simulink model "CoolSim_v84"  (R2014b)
settings: Solver=ode1  StartTime=0.0  StopTime=trun  FixedStep=dtmax  MaxStep=dtmax  MinStep=1e-6  RelTol=1e-4
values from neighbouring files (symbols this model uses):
  aperp_cond = l_cond*gappl_cond - l_cond*densfin_cond*thfin_cond*lfin_cond    (= 0.00397716486616)    [CoolSim_v84_ec_init.m]    (also in CoolSim_v84_mc_init.m)
  apin_txv = 1e-3^2/4*pi    (= 7.85398163397e-07)    [CoolSim_v84_ec_init.m]    (also in CoolSim_v84_mc_init.m)
  area_cabinint = 8.0    (= 8)    [CoolSim_v84_ec_init.m]    (also in CoolSim_v84_mc_init.m)
  area_cabinshell = 4.0    (= 4)    [CoolSim_v84_ec_init.m]    (also in CoolSim_v84_mc_init.m)
  aseat_txv = dball_txv^2/4*pi    (= 7.06858347058e-06)    [CoolSim_v84_ec_init.m]    (also in CoolSim_v84_mc_init.m)
  atop_txv = 400e-6    (= 0.0004)    [CoolSim_v84_ec_init.m]    (also in CoolSim_v84_mc_init.m)
  c08 = -5.8002206e+003    (= -5800.2206)    [CoolSim_v84_ec_init.m]    (also in CoolSim_v84_mc_init.m)
  c09 = 1.3914993    [CoolSim_v84_ec_init.m]    (also in CoolSim_v84_mc_init.m)
  c10 = -4.8640239E-02    (= -0.048640239)    [CoolSim_v84_ec_init.m]    (also in CoolSim_v84_mc_init.m)
  c11 = 4.1764768E-05    (= 4.1764768e-05)    [CoolSim_v84_ec_init.m]    (also in CoolSim_v84_mc_init.m)
  c12 = -1.4452093E-08    (= -1.4452093e-08)    [CoolSim_v84_ec_init.m]    (also in CoolSim_v84_mc_init.m)
  c13 = 6.5459673    [CoolSim_v84_ec_init.m]    (also in CoolSim_v84_mc_init.m)
  c1_comprmech = 0.8728    [CoolSim_v84_ec_init.m]    (also in CoolSim_v84_mc_init.m = 0.9)
  c2_comprmech = 0.1777    [CoolSim_v84_ec_init.m]    (also in CoolSim_v84_mc_init.m = 0)
  cv_air = 719.    (= 719)    [CoolSim_v84_ec_init.m]    (also in CoolSim_v84_mc_init.m)
  deltat = 2e-4    (= 0.0002)    [CoolSim_v84_ec_init.m]    (also in CoolSim_v84_mc_init.m)
  dh_evaptocomp = 0.0    (= 0)    [CoolSim_v84_ec_init.m]    (also in CoolSim_v84_mc_init.m)
  displ_compr = 33e-6    (= 3.3e-05)    [CoolSim_v84_ec_init.m]    (also in CoolSim_v84_mc_init.m = 0.0002)
  dp_blower = [0,  40., 160., 360.]    [CoolSim_v84_ec_init.m]    (also in CoolSim_v84_mc_init.m)
  dp_evaptocomp = 0.0    (= 0)    [CoolSim_v84_ec_init.m]    (also in CoolSim_v84_mc_init.m)
  dpair_cond = 2300.    (= 2300)    [CoolSim_v84_ec_init.m]    (also in CoolSim_v84_mc_init.m)
  dt_evapout = 0.5    [CoolSim_v84_ec_init.m]    (also in CoolSim_v84_mc_init.m)
  dt_thermostat = 0.2    [CoolSim_v84_ec_init.m]    (also in CoolSim_v84_mc_init.m)
  eff_blower = 0.12    [CoolSim_v84_ec_init.m]    (also in CoolSim_v84_mc_init.m)
  eff_fan = 0.15    [CoolSim_v84_ec_init.m]    (also in CoolSim_v84_mc_init.m)
  einitvec_cond1 = 10.*ones(1,nseg_cond1)    [CoolSim_v84_ec_init.m]    (also in CoolSim_v84_mc_init.m)
  einitvec_cond2 = 10.*ones(1,nseg_cond2)    [CoolSim_v84_ec_init.m]    (also in CoolSim_v84_mc_init.m)
  einitvec_evap1 = 10.*ones(1,nseg_evap1)    [CoolSim_v84_ec_init.m]    (also in CoolSim_v84_mc_init.m)
  einitvec_evap2a = 10.*ones(1,nseg_evap2)    [CoolSim_v84_ec_init.m]    (also in CoolSim_v84_mc_init.m)
  einitvec_evap2b = 10.*ones(1,nseg_evap2)    [CoolSim_v84_ec_init.m]    (also in CoolSim_v84_mc_init.m)
  einitvec_evap3 = 10.*ones(1,nseg_evap3)    [CoolSim_v84_ec_init.m]    (also in CoolSim_v84_mc_init.m)
  einitvec_evap4 = 10.*ones(1,nseg_evap4)    [CoolSim_v84_ec_init.m]    (also in CoolSim_v84_mc_init.m)
  f1_blowcontr = -0.7    [CoolSim_v84_ec_init.m]    (also in CoolSim_v84_mc_init.m)
  f1_comprcontr = -0.02    [CoolSim_v84_ec_init.m]    (also in CoolSim_v84_mc_init.m)
  f2_blowcontr = 0.005    [CoolSim_v84_ec_init.m]    (also in CoolSim_v84_mc_init.m)
  f2_comprcontr = 1./6.    (= 0.166666666667)    [CoolSim_v84_ec_init.m]    (also in CoolSim_v84_mc_init.m)
  fp_txv = (psetbulb_txv - pset_txv)*atop_txv - 15e5*aseat_txv    [CoolSim_v84_ec_init.m]    (also in CoolSim_v84_mc_init.m)
  h_lookuphvsps = h1    [CoolSim_v84_ec_init.m]    (also in CoolSim_v84_mc_init.m)
  hmax_heater = 8000.    (= 8000)    [CoolSim_v84_ec_init.m]    (also in CoolSim_v84_mc_init.m)
  htin_enginecomp = 0.0    (= 0)    [CoolSim_v84_ec_init.m]    (also in CoolSim_v84_mc_init.m; point_ec01.m; point_mc01.m)
  htin_solarintvstime = [htin_solarint htin_solarint]    [CoolSim_v84_ec_init.m]    (also in CoolSim_v84_mc_init.m; point_ec01.m = [300. 300.]; point_mc01.m = [300. 300.])
  htin_solarshellvstime = [htin_solarshell htin_solarshell]    [CoolSim_v84_ec_init.m]    (also in CoolSim_v84_mc_init.m; point_ec01.m = [1000. 1000.]; point_mc01.m = [1000. 1000.])
  htrans_cabinint = 25.    (= 25)    [CoolSim_v84_ec_init.m]    (also in CoolSim_v84_mc_init.m)
  htrans_cabinshell = 15.    (= 15)    [CoolSim_v84_ec_init.m]    (also in CoolSim_v84_mc_init.m)
  ifmech = 0.0    (= 0)    [CoolSim_v84_ec_init.m]    (also in CoolSim_v84_mc_init.m = 1)
  iinitvec_cond1 = 0.0*ones(1,nseg_cond1+1)    [CoolSim_v84_ec_init.m]    (also in CoolSim_v84_mc_init.m)
  iinitvec_cond2 = 0.0*ones(1,nseg_cond2+1)    [CoolSim_v84_ec_init.m]    (also in CoolSim_v84_mc_init.m)
  iinitvec_evap1 = 0.0*ones(1,nseg_evap1+1)    [CoolSim_v84_ec_init.m]    (also in CoolSim_v84_mc_init.m)
  iinitvec_evap2a = 0.0*ones(1,nseg_evap2+1)    [CoolSim_v84_ec_init.m]    (also in CoolSim_v84_mc_init.m)
  iinitvec_evap2b = 0.0*ones(1,nseg_evap2+1)    [CoolSim_v84_ec_init.m]    (also in CoolSim_v84_mc_init.m)
  iinitvec_evap3 = 0.0*ones(1,nseg_evap3+1)    [CoolSim_v84_ec_init.m]    (also in CoolSim_v84_mc_init.m)
  iinitvec_evap4 = 0.0*ones(1,nseg_evap4+1)    [CoolSim_v84_ec_init.m]    (also in CoolSim_v84_mc_init.m)
  init_memrestart = 2250.    (= 2250)    [CoolSim_v84_ec_init.m]    (also in CoolSim_v84_mc_init.m; reinit.m = memrestart(n,2))
  init_picontr1 = 0.23    [CoolSim_v84_ec_init.m]    (also in CoolSim_v84_mc_init.m; reinit.m = picontr1(n,2))
  init_picontr2 = 0.32    [CoolSim_v84_ec_init.m]    (also in CoolSim_v84_mc_init.m; reinit.m = picontr2(n,2))
  iseff_rpm_pr = [0.650   0.728   0.717   0.655   0.569;     0.570   0.682   0.700   0.637   0.536;     0.460   0.590   0.650   0.600   0.493;     0.290   0.496   0.618   0.575   0.450]    [CoolSim_v84_ec_init.m]    (also in CoolSim_v84_mc_init.m = [0.8490    0.8490    0.7829    0.7409    0.7065    0.6802   )
  k_cabinleakin = 1e-4    (= 0.0001)    [CoolSim_v84_ec_init.m]    (also in CoolSim_v84_mc_init.m)
  k_cabinleakout = 4e-4    (= 0.0004)    [CoolSim_v84_ec_init.m]    (also in CoolSim_v84_mc_init.m)
  k_ram = 0.1    [CoolSim_v84_ec_init.m]    (also in CoolSim_v84_mc_init.m)
  l_cabinsurf = 2.0    (= 2)    [CoolSim_v84_ec_init.m]    (also in CoolSim_v84_mc_init.m)
  md_comprmax = rpm_max/60.*displ_compr*0.975*27.8    (= 0.10435425)    [CoolSim_v84_ec_init.m]    (also in CoolSim_v84_mc_init.m = 0.63245)
  minitvec_cond1 = 1e-4*ones(1,nseg_cond1)    [CoolSim_v84_ec_init.m]    (also in CoolSim_v84_mc_init.m)
  minitvec_cond2 = 1e-4*ones(1,nseg_cond2)    [CoolSim_v84_ec_init.m]    (also in CoolSim_v84_mc_init.m)
  minitvec_evap1 = 1e-4*ones(1,nseg_evap1)    [CoolSim_v84_ec_init.m]    (also in CoolSim_v84_mc_init.m)
  minitvec_evap2a = 1e-4*ones(1,nseg_evap2)    [CoolSim_v84_ec_init.m]    (also in CoolSim_v84_mc_init.m)
  minitvec_evap2b = 1e-4*ones(1,nseg_evap2)    [CoolSim_v84_ec_init.m]    (also in CoolSim_v84_mc_init.m)
  minitvec_evap3 = 1e-4*ones(1,nseg_evap3)    [CoolSim_v84_ec_init.m]    (also in CoolSim_v84_mc_init.m)
  minitvec_evap4 = 1e-4*ones(1,nseg_evap4)    [CoolSim_v84_ec_init.m]    (also in CoolSim_v84_mc_init.m)
  mrefr_outrate = 0.2    [CoolSim_v84_ec_init.m]    (also in CoolSim_v84_mc_init.m)
  mrefr_targ = 0.48    [CoolSim_v84_ec_init.m]    (also in CoolSim_v84_mc_init.m)
  nc1 = 35.    (= 35)    [CoolSim_v84_ec_init.m]    (also in CoolSim_v84_mc_init.m)
  nc2 = 9.0    (= 9)    [CoolSim_v84_ec_init.m]    (also in CoolSim_v84_mc_init.m)
  ne1 = 7.    (= 7)    [CoolSim_v84_ec_init.m]    (also in CoolSim_v84_mc_init.m)
  ne2a = 5.    (= 5)    [CoolSim_v84_ec_init.m]    (also in CoolSim_v84_mc_init.m)
  ne2b = 15.    (= 15)    [CoolSim_v84_ec_init.m]    (also in CoolSim_v84_mc_init.m)
  ne3 = 12.    (= 12)    [CoolSim_v84_ec_init.m]    (also in CoolSim_v84_mc_init.m)
  ne4 = 15.    (= 15)    [CoolSim_v84_ec_init.m]    (also in CoolSim_v84_mc_init.m)
  onoff_fanonoffvstime = [1  1]    [CoolSim_v84_ec_init.m]    (also in CoolSim_v84_mc_init.m; point_ec01.m; point_mc01.m)
  onoffinit_cabin = 1.0    (= 1)    [CoolSim_v84_ec_init.m]    (also in CoolSim_v84_mc_init.m; reinit.m = onoff_cabin(n,2))
  onoffinit_evap = 1.0    (= 1)    [CoolSim_v84_ec_init.m]    (also in CoolSim_v84_mc_init.m; reinit.m = onoff_evap(n,2))
  p_ambient = 1.013e5    (= 101300)    [CoolSim_v84_ec_init.m]    (also in CoolSim_v84_mc_init.m)
  p_ambvstime = [p_ambient p_ambient]    [CoolSim_v84_ec_init.m]    (also in CoolSim_v84_mc_init.m; point_ec01.m = [101300. 101300.]; point_mc01.m = [101300. 101300.])
  p_lookup_tsatvsp = psat*1e5    [CoolSim_v84_ec_init.m]    (also in CoolSim_v84_mc_init.m)
  r_h2o = 461.5043    [CoolSim_v84_ec_init.m]    (also in CoolSim_v84_mc_init.m)
  rair = 287.    (= 287)    [CoolSim_v84_ec_init.m]    (also in CoolSim_v84_mc_init.m)
  rate_txv = 35e3    (= 35000)    [CoolSim_v84_ec_init.m]    (also in CoolSim_v84_mc_init.m)
  ratio_compr = 1.37    [CoolSim_v84_ec_init.m]    (also in CoolSim_v84_mc_init.m)
  rh_ambvstime = [rh_ambient rh_ambient]    [CoolSim_v84_ec_init.m]    (also in CoolSim_v84_mc_init.m; point_ec01.m = [50. 50.]; point_mc01.m = [50. 50.])
  rpm_max = 7000.    (= 7000)    [CoolSim_v84_ec_init.m]    (also in CoolSim_v84_mc_init.m)
  rpm_minmaxrat = 1500./7000.    (= 0.214285714286)    [CoolSim_v84_ec_init.m]    (also in CoolSim_v84_mc_init.m)
  rpm_rpmvstime = [1600,  1600]    [CoolSim_v84_ec_init.m]    (also in CoolSim_v84_mc_init.m; point_mc01.m)
  rpm_switchoff = rpm_max*rpm_minmaxrat*1.01    (= 1515)    [CoolSim_v84_ec_init.m]    (also in CoolSim_v84_mc_init.m)
  s_txv = 0.8e-3    (= 0.0008)    [CoolSim_v84_ec_init.m]    (also in CoolSim_v84_mc_init.m)
  scfm_blower = [0, 100., 200., 300.]    [CoolSim_v84_ec_init.m]    (also in CoolSim_v84_mc_init.m)
  set_steadystate = 0.0    (= 0)    [CoolSim_v84_ec_init.m]    (also in CoolSim_v84_mc_init.m)
  setting_blend = 0.0    (= 0)    [CoolSim_v84_ec_init.m]    (also in CoolSim_v84_mc_init.m; point_mc01.m)
  setting_blower = 3.0    (= 3)    [CoolSim_v84_ec_init.m]    (also in CoolSim_v84_mc_init.m; point_mc01.m)
  setting_recirc = -1.0    (= -1)    [CoolSim_v84_ec_init.m]    (also in CoolSim_v84_mc_init.m; point_mc01.m = 0.95)
  shape_cabinsurf = 0.5    [CoolSim_v84_ec_init.m]    (also in CoolSim_v84_mc_init.m)
  smin_txv = 1e-6    (= 1e-06)    [CoolSim_v84_ec_init.m]    (also in CoolSim_v84_mc_init.m)
  t_ambvstime = [t_ambient t_ambient]    [CoolSim_v84_ec_init.m]    (also in CoolSim_v84_mc_init.m; point_ec01.m = [303.16 303.16]; point_mc01.m = [303.16 303.16])
  t_lookup_tsatvsp = t1    [CoolSim_v84_ec_init.m]    (also in CoolSim_v84_mc_init.m)
  tairevapout_limit = 274.    (= 274)    [CoolSim_v84_ec_init.m]    (also in CoolSim_v84_mc_init.m)
  tairin_cond = 303.16    [CoolSim_v84_ec_init.m]    (also in CoolSim_v84_mc_init.m; point_ec01.m; point_mc01.m)
  tbulbinit_txv = 273.0    (= 273)    [CoolSim_v84_ec_init.m]    (also in CoolSim_v84_mc_init.m; reinit.m = tbulb_txv(n,2))
  tchar_txv = 0.1    [CoolSim_v84_ec_init.m]    (also in CoolSim_v84_mc_init.m)
  tdel_cycling = 5.0    (= 5)    [CoolSim_v84_ec_init.m]    (also in CoolSim_v84_mc_init.m)
  tdelinit_cycling = 1.0    (= 1)    [CoolSim_v84_ec_init.m]    (also in CoolSim_v84_mc_init.m; reinit.m = tdel_cycling1(n,2))
  tevap_target = 273.16+3.0    (= 276.16)    [CoolSim_v84_ec_init.m]    (also in CoolSim_v84_mc_init.m)
  thmass_cabinint = 2e5    (= 200000)    [CoolSim_v84_ec_init.m]    (also in CoolSim_v84_mc_init.m)
  thmass_cabinshell = 1e5    (= 100000)    [CoolSim_v84_ec_init.m]    (also in CoolSim_v84_mc_init.m)
  time0 = 0.0    (= 0)    [CoolSim_v84_ec_init.m]    (also in CoolSim_v84_mc_init.m; reinit.m = time11(n,2))
  time_ambvstime = [0 1e5]    [CoolSim_v84_ec_init.m]    (also in CoolSim_v84_mc_init.m; point_ec01.m; point_mc01.m)
  time_fanonoffvstime = [0 1e5]    [CoolSim_v84_ec_init.m]    (also in CoolSim_v84_mc_init.m; point_ec01.m; point_mc01.m)
  time_rpmvstime = [0,    10000]    [CoolSim_v84_ec_init.m]    (also in CoolSim_v84_mc_init.m; point_mc01.m)
  time_solarintvstime = [0 1e5]    [CoolSim_v84_ec_init.m]    (also in CoolSim_v84_mc_init.m; point_ec01.m; point_mc01.m)
  time_solarshellvstime = [0 1e5]    [CoolSim_v84_ec_init.m]    (also in CoolSim_v84_mc_init.m; point_ec01.m; point_mc01.m)
  time_velvstime = [0 1e5]    [CoolSim_v84_ec_init.m]    (also in CoolSim_v84_mc_init.m; point_ec01.m; point_mc01.m)
  tinit_cabinint = 313.16    [CoolSim_v84_ec_init.m]    (also in CoolSim_v84_mc_init.m; point_ec01.m; point_mc01.m; reinit.m = t_cabinint(n,2))
  tinit_cabinshell = 308.16    [CoolSim_v84_ec_init.m]    (also in CoolSim_v84_mc_init.m; point_ec01.m; point_mc01.m; reinit.m = t_cabinshell(n,2))
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undefined symbols (not defined in the file or in its folder): nseg
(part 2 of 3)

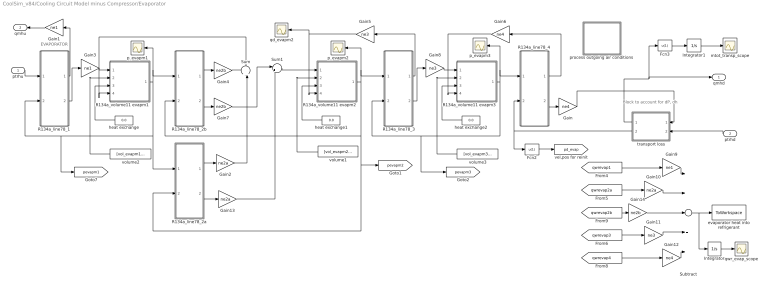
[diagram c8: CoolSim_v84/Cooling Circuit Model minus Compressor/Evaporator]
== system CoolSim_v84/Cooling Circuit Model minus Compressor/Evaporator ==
  note: EVAPORATOR
  note: Block to account for dP, dh
  ptrhu : Inport
  ptrhd : Inport  Port=2
  Fcn2 : Fcn  Expr=u(1)
  Fcn3 : Fcn  Expr=u(1)
  Gain : Gain  Gain=ne4
  Gain1 : Gain  Gain=ne1
  Gain10 : Gain  Gain=ne2a
  Gain11 : Gain  Gain=ne3
  Gain12 : Gain  Gain=ne4
  Gain13 : Gain  Gain=ne2a
  Gain14 : Gain  Gain=ne2b
  Gain2 : Gain  Gain=ne2a
  Gain3 : Gain  Gain=ne1
  Gain4 : Gain  Gain=ne2b
  Gain5 : Gain  Gain=ne3
  Gain6 : Gain  Gain=ne4
  Gain7 : Gain  Gain=ne2b
  Gain8 : Gain  Gain=ne3
  Gain9 : Gain  Gain=ne1
  Integrator : Integrator
  Integrator1 : Integrator
  R134a_line78_1 : Subsystem
  R134a_line78_2a : Subsystem
  R134a_line78_2b : Subsystem
  R134a_line78_3 : Subsystem
  R134a_line78_4 : Subsystem
  R134a_volume11 evapm1 : Subsystem
  R134a_volume11 evapm2 : Subsystem
  R134a_volume11 evapm3 : Subsystem
  Subtract : Sum  Inputs=+++++
  Sum : Sum  Inputs=++|
  Sum1 : Sum  Inputs=|++
  evaporator heat into refrigerant : ToWorkspace  VariableName=qwr_evap  SampleTime=-1
  heat exchange : Constant  Value=0.0
  heat exchange1 : Constant  Value=0.0
  heat exchange2 : Constant  Value=0.0
  mtot_transp_scope : Scope
  p_evapm1 : Scope
  p_evapm2 : Scope
  p_evapm3 : Scope
  process outgoing air conditions : Subsystem
  qd_evapm2 : Scope
  qwr_evap_scope : Scope
  transport loss : Subsystem
  volume1 : Constant  Value=[vol_evapm2, 0]
  volume2 : Constant  Value=[vol_evapm1, 0]
  volume3 : Constant  Value=[vol_evapm3, 0]
  qmhd : Outport
  qmhu : Outport  Port=2
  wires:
  Gain14/1 -> Subtract/3
  [qwrevap2b] -> Gain14/1
  Gain12/1 -> Subtract/5
  [qwrevap4] -> Gain12/1
  Gain11/1 -> Subtract/4
  Gain13/1 -> Sum1/2
  R134a_line78_2a/2(qmhd) -> Gain13/1
  Gain7/1 -> Sum1/1
  Gain2/1 -> Sum/2
  Gain4/1 -> Sum/1
  R134a_line78_2b/1(qmhu) -> Gain4/1
  Sum/1 -> R134a_volume11 evapm1/4(qd)
  R134a_line78_2a/1(qmhu) -> Gain2/1
  Gain10/1 -> Subtract/2
  Gain9/1 -> Subtract/1
  Gain8/1 -> R134a_volume11 evapm3/1(qu)
  Sum1/1 -> R134a_volume11 evapm2/1(qu)
  Gain6/1 -> R134a_volume11 evapm3/4(qd)
  Gain5/1 -> R134a_volume11 evapm2/4(qd), qd_evapm2/1
  Gain3/1 -> R134a_volume11 evapm1/1(qu)
  Subtract/1 -> evaporator heat into refrigerant/1, Integrator/1
  [qwrevap3] -> Gain11/1
  [qwrevap2a] -> Gain10/1
  [qwrevap1] -> Gain9/1
  Gain1/1 -> qmhu/1
  R134a_line78_4/2(qmhd) -> Gain/1
  R134a_line78_4/1(qmhu) -> Gain6/1
  R134a_volume11 evapm3/1(ptrh_mix) -> p_evapm3/1, R134a_line78_4/1(pTrhu), R134a_line78_3/2(pTrhd), [pevapm3]
  volume3/1 -> R134a_volume11 evapm3/2("V, dVdt")
  heat exchange2/1 -> R134a_volume11 evapm3/3(Hout)
  R134a_line78_3/2(qmhd) -> Gain8/1
  R134a_line78_3/1(qmhu) -> Gain5/1
  R134a_volume11 evapm2/1(ptrh_mix) -> R134a_line78_2b/2(pTrhd), R134a_line78_2a/2(pTrhd), [pevapm2], p_evapm2/1, R134a_line78_3/1(pTrhu)
  volume1/1 -> R134a_volume11 evapm2/2("V, dVdt")
  heat exchange1/1 -> R134a_volume11 evapm2/3(Hout)
  R134a_line78_2b/2(qmhd) -> Gain7/1
  R134a_volume11 evapm1/1(ptrh_mix) -> R134a_line78_2a/1(pTrhu), R134a_line78_1/2(pTrhd), [pevapm1], R134a_line78_2b/1(pTrhu), p_evapm1/1
  volume2/1 -> R134a_volume11 evapm1/2("V, dVdt")
  heat exchange/1 -> R134a_volume11 evapm1/3(Hout)
  ptrhu/1 -> R134a_line78_1/1(pTrhu)
  R134a_line78_1/1(qmhu) -> Gain1/1
  R134a_line78_1/2(qmhd) -> Gain3/1
  transport loss/1(qd) -> qmhd/1, Fcn3/1
  Gain/1 -> transport loss/1(qu)
  ptrhd/1 -> transport loss/2(pd)
  transport loss/2(pu) -> Fcn2/1, R134a_line78_4/2(pTrhd)
  Fcn2/1 -> [pd_evap]
  Integrator/1 -> qwr_evap_scope/1
  Integrator1/1 -> mtot_transp_scope/1
  Fcn3/1 -> Integrator1/1

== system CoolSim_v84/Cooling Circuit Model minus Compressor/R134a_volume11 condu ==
  note: p, T, rho, h vapor phase
  note: p, T, rho, h liquid phase
  note: number of messages
  note: p, T, rho, h mixture
  qu : Inport
  "V, dVdt" : Inport  Port=2
  Hout : Inport  Port=3
  qd : Inport  Port=4
  S-Function : S-Function  FunctionName=R134a_volume11  Parameters=vol0, p0, tmp0, hspec0, lvf0, relerr, itmx, dgns  EnableBusSupport=off
  Terminator : Terminator
  Terminator1 : Terminator
  Terminator2 : Terminator
  ptrh_mix : Outport
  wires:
  S-Function/4 -> [lvfcondu]
  S-Function/3 -> Terminator1/1
  S-Function/2 -> Terminator/1
  S-Function/5 -> Terminator2/1
  qd/1 -> S-Function/4
  Hout/1 -> S-Function/3
  "V, dVdt"/1 -> S-Function/2
  S-Function/1 -> ptrh_mix/1
  qu/1 -> S-Function/1

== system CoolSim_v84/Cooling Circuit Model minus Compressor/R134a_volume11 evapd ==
  note: p, T, rho, h vapor phase
  note: p, T, rho, h liquid phase
  note: number of messages
  note: p, T, rho, h mixture
  qu : Inport
  "V, dVdt" : Inport  Port=2
  Hout : Inport  Port=3
  qd : Inport  Port=4
  S-Function : S-Function  FunctionName=R134a_volume11  Parameters=vol0, p0, tmp0, hspec0, lvf0, relerr, itmx, dgns  EnableBusSupport=off
  Terminator : Terminator
  Terminator1 : Terminator
  Terminator2 : Terminator
  ptrh_mix : Outport
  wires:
  S-Function/4 -> [lvfevapd]
  S-Function/3 -> Terminator1/1
  S-Function/2 -> Terminator/1
  S-Function/5 -> Terminator2/1
  qd/1 -> S-Function/4
  Hout/1 -> S-Function/3
  "V, dVdt"/1 -> S-Function/2
  S-Function/1 -> ptrh_mix/1
  qu/1 -> S-Function/1

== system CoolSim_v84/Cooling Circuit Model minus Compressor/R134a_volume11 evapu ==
  note: p, T, rho, h vapor phase
  note: p, T, rho, h liquid phase
  note: number of messages
  note: p, T, rho, h mixture
  qu : Inport
  "V, dVdt" : Inport  Port=2
  Hout : Inport  Port=3
  qd : Inport  Port=4
  S-Function : S-Function  FunctionName=R134a_volume11  Parameters=vol0, p0, tmp0, hspec0, lvf0, relerr, itmx, dgns  EnableBusSupport=off
  Terminator : Terminator
  Terminator1 : Terminator
  Terminator2 : Terminator
  ptrh_mix : Outport
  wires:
  S-Function/4 -> [lvfevapu]
  S-Function/3 -> Terminator1/1
  S-Function/2 -> Terminator/1
  S-Function/5 -> Terminator2/1
  qd/1 -> S-Function/4
  Hout/1 -> S-Function/3
  "V, dVdt"/1 -> S-Function/2
  S-Function/1 -> ptrh_mix/1
  qu/1 -> S-Function/1

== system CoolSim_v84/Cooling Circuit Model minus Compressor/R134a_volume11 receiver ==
  note: p, T, rho, h vapor phase
  note: p, T, rho, h liquid phase
  note: number of messages
  note: p,T,rho,h mixture
  qu : Inport
  "V, dVdt" : Inport  Port=2
  Hout : Inport  Port=3
  qd : Inport  Port=4
  Divide : Product  Inputs=**
  Divide1 : Product  Inputs=**
  Mux : Mux  Inputs=2
  S-Function : S-Function  FunctionName=R134a_volume11  Parameters=vol0, p0, tmp0, hspec0, lvf0, relerr, itmx, dgns  EnableBusSupport=off
  Sum : Sum  Inputs=|++
  Sum1 : Sum  Inputs=|+-
  Terminator : Terminator
  Terminator1 : Terminator
  Terminator2 : Terminator
  enthalpy : Fcn  Expr=u(4)
  target system refrigerant mass : Constant  Value=mrefr_targ
  target system refrigerant mass1 : Constant  Value=mrefr_outrate
  ptrh_mix : Outport
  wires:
  S-Function/4 -> [lvfreceiver]
  S-Function/3 -> Terminator1/1
  S-Function/2 -> Terminator/1
  S-Function/5 -> Terminator2/1
  Hout/1 -> S-Function/3
  "V, dVdt"/1 -> S-Function/2
  S-Function/1 -> ptrh_mix/1, enthalpy/1
  qu/1 -> S-Function/1
  Sum/1 -> S-Function/4
  qd/1 -> Sum/1
  [mrefr] -> Sum1/1
  target system refrigerant mass/1 -> Sum1/2
  Sum1/1 -> Divide/1
  target system refrigerant mass1/1 -> Divide/2
  Mux/1 -> Sum/2
  Divide/1 -> Mux/1, Divide1/1
  Divide1/1 -> Mux/2
  enthalpy/1 -> Divide1/2

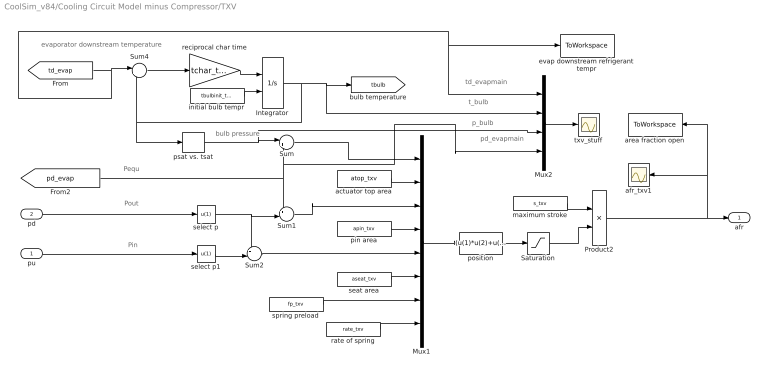
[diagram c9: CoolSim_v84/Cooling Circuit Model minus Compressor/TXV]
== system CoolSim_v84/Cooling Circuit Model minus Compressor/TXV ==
  note: evaporator downstream temperature
  note: bulb pressure
  note: pd_evapmain
  note: p_bulb
  note: t_bulb
  note: td_evapmain
  note: Pequ
  note: Pout
  note: Pin
  pu : Inport
  pd : Inport  Port=2
  Integrator : Integrator  InitialConditionSource=external  InitialCondition=tbulbinit_txv
  Mux1 : Mux  Inputs=8
  Mux2 : Mux
  Product2 : Product  Inputs=/*
  Saturation : Saturate  UpperLimit=s_txv  LowerLimit=smin_txv
  Sum : Sum  Inputs=|+-
  Sum1 : Sum  Inputs=+-|
  Sum2 : Sum  Inputs=+-|
  Sum4 : Sum  Inputs=|+-
  actuator top area : Constant  Value=atop_txv
  afr_txv1 : Scope
  area fraction open : ToWorkspace  VariableName=afr_txv  SampleTime=-1
  evap downstream refrigerant tempr : ToWorkspace  VariableName=tdevap  SampleTime=-1
  initial bulb tempr : Constant  Value=tbulbinit_txv
  maximum stroke : Constant  Value=s_txv
  pin area : Constant  Value=apin_txv
  position : Fcn  Expr=(u(1)*u(2)+u(3)*u(4)+u(5)*u(6)-u(7))/u(8)
  psat vs. tsat : Lookup_n-D  NumberOfTableDimensions=1  BreakpointsForDimension1=t_lookup_tsatvsp  Table=p_lookup_tsatvsp  RndMeth=Simplest
  rate of spring : Constant  Value=rate_txv
  reciprocal char time : Gain  Gain=tchar_txv
  seat area : Constant  Value=aseat_txv
  select p : Fcn  Expr=u(1)
  select p1 : Fcn  Expr=u(1)
  spring preload : Constant  Value=fp_txv
  txv_stuff : Scope
  afr : Outport
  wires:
  initial bulb tempr/1 -> Integrator/2
  select p1/1 -> Sum2/2
  select p/1 -> Sum2/1, Sum1/2
  maximum stroke/1 -> Product2/1
  Product2/1 -> afr/1, afr_txv1/1, area fraction open/1
  reciprocal char time/1 -> Integrator/1
  Sum4/1 -> reciprocal char time/1
  psat vs. tsat/1 -> Sum/1, Mux2/3
  Mux1/1 -> position/1
  seat area/1 -> Mux1/6
  Sum2/1 -> Mux1/5
  pu/1 -> select p1/1
  pin area/1 -> Mux1/4
  Sum1/1 -> Mux1/3
  pd/1 -> select p/1
  actuator top area/1 -> Mux1/2
  Sum/1 -> Mux1/1
  Integrator/1 -> Sum4/2, psat vs. tsat/1, [tbulb], Mux2/2
  [pd_evap] -> Sum1/1, Sum/2, Mux2/4
  [td_evap] -> Sum4/1, Mux2/1, evap downstream refrigerant tempr/1
  Mux2/1 -> txv_stuff/1
  spring preload/1 -> Mux1/7
  rate of spring/1 -> Mux1/8
  position/1 -> Saturation/1
  Saturation/1 -> Product2/2

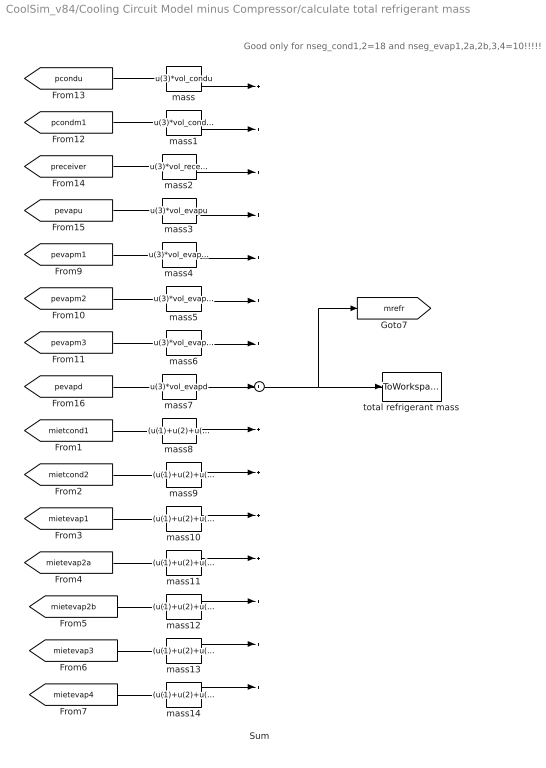
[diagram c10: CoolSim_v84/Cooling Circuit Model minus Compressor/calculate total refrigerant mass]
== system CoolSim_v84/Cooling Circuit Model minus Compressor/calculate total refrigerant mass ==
  note: Good only for nseg_cond1,2=18 and nseg_evap1,2a,2b,3,4=10!!!!!
  Sum : Sum  Inputs=+++++++++++++++
  mass : Fcn  Expr=u(3)*vol_condu
  mass1 : Fcn  Expr=u(3)*vol_condm1
  mass10 : Fcn  Expr=(u(1)+u(2)+u(3)+u(4)+u(5)+u(6)+u(7)+u(8)+u(9)+u(10))*ne1
  mass11 : Fcn  Expr=(u(1)+u(2)+u(3)+u(4)+u(5)+u(6)+u(7)+u(8)+u(9)+u(10))*ne2a
  mass12 : Fcn  Expr=(u(1)+u(2)+u(3)+u(4)+u(5)+u(6)+u(7)+u(8)+u(9)+u(10))*ne2b
  mass13 : Fcn  Expr=(u(1)+u(2)+u(3)+u(4)+u(5)+u(6)+u(7)+u(8)+u(9)+u(10))*ne3
  mass14 : Fcn  Expr=(u(1)+u(2)+u(3)+u(4)+u(5)+u(6)+u(7)+u(8)+u(9)+u(10))*ne4
  mass2 : Fcn  Expr=u(3)*vol_receiver
  mass3 : Fcn  Expr=u(3)*vol_evapu
  mass4 : Fcn  Expr=u(3)*vol_evapm1
  mass5 : Fcn  Expr=u(3)*vol_evapm2
  mass6 : Fcn  Expr=u(3)*vol_evapm3
  mass7 : Fcn  Expr=u(3)*vol_evapd
  mass8 : Fcn  Expr=(u(1)+u(2)+u(3)+u(4)+u(5)+u(6)+u(7)+u(8)+u(9)+u(10)+u(11)+u(12)+u(13)+u(14)+u(15)+u(16)+u(17)+u(18))*nc1
  mass9 : Fcn  Expr=(u(1)+u(2)+u(3)+u(4)+u(5)+u(6)+u(7)+u(8)+u(9)+u(10)+u(11)+u(12)+u(13)+u(14)+u(15)+u(16)+u(17)+u(18))*nc2
  total refrigerant mass : ToWorkspace  VariableName=mtotrefr  SampleTime=-1
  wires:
  [pcondu] -> mass/1
  [pevapd] -> mass7/1
  [pevapm3] -> mass6/1
  [pevapm2] -> mass5/1
  [pevapm1] -> mass4/1
  [pevapu] -> mass3/1
  [preceiver] -> mass2/1
  [pcondm1] -> mass1/1
  [mietcond1] -> mass8/1
  [mietcond2] -> mass9/1
  [mietevap1] -> mass10/1
  [mietevap2a] -> mass11/1
  [mietevap2b] -> mass12/1
  [mietevap3] -> mass13/1
  [mietevap4] -> mass14/1
  mass/1 -> Sum/1
  mass1/1 -> Sum/2
  mass2/1 -> Sum/3
  mass3/1 -> Sum/4
  mass4/1 -> Sum/5
  mass5/1 -> Sum/6
  mass6/1 -> Sum/7
  mass7/1 -> Sum/8
  mass8/1 -> Sum/9
  mass9/1 -> Sum/10
  mass10/1 -> Sum/11
  mass11/1 -> Sum/12
  mass12/1 -> Sum/13
  mass13/1 -> Sum/14
  mass14/1 -> Sum/15
  Sum/1 -> total refrigerant mass/1, [mrefr]

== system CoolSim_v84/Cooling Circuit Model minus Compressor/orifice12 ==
  pTrhu : Inport
  afrac : Inport  Port=2
  pTrhd : Inport  Port=3
  S-Function : S-Function  FunctionName=orifice13  Parameters=amax, cdfw, cdbk, kcd1, kcd2, kcd3, kcd4, dgns  EnableBusSupport=off
  Terminator : Terminator
  qmh : Outport
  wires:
  S-Function/2 -> Terminator/1
  pTrhd/1 -> S-Function/3
  S-Function/1 -> qmh/1
  afrac/1 -> S-Function/2
  pTrhu/1 -> S-Function/1

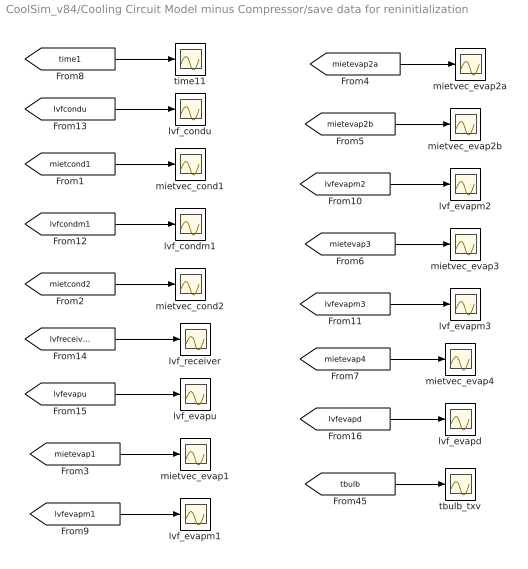
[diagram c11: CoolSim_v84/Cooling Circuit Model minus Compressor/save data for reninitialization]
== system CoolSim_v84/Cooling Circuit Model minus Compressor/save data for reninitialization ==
  lvf_condm1 : Scope
  lvf_condu : Scope
  lvf_evapd : Scope
  lvf_evapm1 : Scope
  lvf_evapm2 : Scope
  lvf_evapm3 : Scope
  lvf_evapu : Scope
  lvf_receiver : Scope
  mietvec_cond1 : Scope
  mietvec_cond2 : Scope
  mietvec_evap1 : Scope
  mietvec_evap2a : Scope
  mietvec_evap2b : Scope
  mietvec_evap3 : Scope
  mietvec_evap4 : Scope
  tbulb_txv : Scope
  time11 : Scope
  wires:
  [lvfevapm2] -> lvf_evapm2/1
  [lvfevapm3] -> lvf_evapm3/1
  [lvfevapm1] -> lvf_evapm1/1
  [lvfcondm1] -> lvf_condm1/1
  [mietcond1] -> mietvec_cond1/1
  [mietcond2] -> mietvec_cond2/1
  [mietevap4] -> mietvec_evap4/1
  [mietevap3] -> mietvec_evap3/1
  [mietevap2b] -> mietvec_evap2b/1
  [mietevap2a] -> mietvec_evap2a/1
  [mietevap1] -> mietvec_evap1/1
  [lvfcondu] -> lvf_condu/1
  [lvfreceiver] -> lvf_receiver/1
  [lvfevapu] -> lvf_evapu/1
  [lvfevapd] -> lvf_evapd/1
  [tbulb] -> tbulb_txv/1
  [time1] -> time11/1

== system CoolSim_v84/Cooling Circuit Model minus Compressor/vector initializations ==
  initialization vectors : Constant  Value=[minitvec_cond1, iinitvec_cond1, einitvec_cond1, twinitvec_cond1]
  initialization vectors - evaporator pass 1 : Constant  Value=[minitvec_evap1, iinitvec_evap1, einitvec_evap1, twinitvec_evap1]
  initialization vectors1 : Constant  Value=[minitvec_cond2, iinitvec_cond2, einitvec_cond2, twinitvec_cond2]
  initialization vectors2 : Constant  Value=[minitvec_evap2b, iinitvec_evap2b, einitvec_evap2b, twinitvec_evap2b]
  initialization vectors3 : Constant  Value=[minitvec_evap2a, iinitvec_evap2a, einitvec_evap2a, twinitvec_evap2a]
  initialization vectors4 : Constant  Value=[minitvec_evap3, iinitvec_evap3, einitvec_evap3, twinitvec_evap3]
  initialization vectors5 : Constant  Value=[minitvec_evap4, iinitvec_evap4, einitvec_evap4, twinitvec_evap4]
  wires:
  initialization vectors - evaporator pass 1/1 -> [initevap1]
  initialization vectors3/1 -> [initevap2a]
  initialization vectors2/1 -> [initevap2b]
  initialization vectors4/1 -> [initevap3]
  initialization vectors5/1 -> [initevap4]
  initialization vectors1/1 -> [initcond2]
  initialization vectors/1 -> [initcond1]

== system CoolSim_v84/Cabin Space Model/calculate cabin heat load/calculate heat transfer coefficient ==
  note: heat transfer coeff
  note: Incropera, Eq. 7-43
  vveh : Inport
  Ingth : Inport  Port=2
  amb : Inport  Port=3
  Lookup therm.conductivity : Lookup_n-D  NumberOfTableDimensions=1  BreakpointsForDimension1=[222.22, 249.99, 277.77, 305.55, 333.33, 361.10]  Table=[20.42e-3, 22.50e-3, 24.75e-3, 27.00e-3, 29.08e-3, 31.15e-3]  RndMeth=Simplest
  Lookup viscosity : Lookup_n-D  NumberOfTableDimensions=1  BreakpointsForDimension1=[222.22, 249.99, 277.77, 305.55, 333.33, 361.10]  Table=[1.488e-5, 1.622e-5, 1.756e-5, 1.875e-5, 2.009e-5, 2.128e-5]  RndMeth=Simplest
  Mux : Mux  Inputs=2
  Product : Product  Inputs=**/
  Product1 : Product  Inputs=**/*
  air Prandtl num : Constant  Value=0.72
  calc avg Nuss : Fcn  Expr=0.037*u(2)^0.8*u(1)^0.3333
  calc rho : Fcn  Expr=u(1)/rair/u(2)
  select tempr : Fcn  Expr=u(2)
  h : Outport
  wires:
  Product/1 -> h/1
  amb/1 -> select tempr/1, calc rho/1
  select tempr/1 -> Lookup viscosity/1, Lookup therm.conductivity/1
  Ingth/1 -> Product1/4, Product/3
  Lookup viscosity/1 -> Product1/3
  calc rho/1 -> Product1/2
  vveh/1 -> Product1/1
  Product1/1 -> Mux/2
  air Prandtl num/1 -> Mux/1
  Mux/1 -> calc avg Nuss/1
  Lookup therm.conductivity/1 -> Product/1
  calc avg Nuss/1 -> Product/2

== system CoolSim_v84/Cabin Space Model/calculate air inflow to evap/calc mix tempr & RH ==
  press : Inport
  enth : Inport  Port=2
  AH : Inport  Port=3
  Demux : Demux  Outputs=3
  Mux3 : Mux  Inputs=3
  S-Function : S-Function  FunctionName=tempr_from_phw  EnableBusSupport=off
  Terminator : Terminator
  tempr : Outport
  RH : Outport  Port=2
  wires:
  press/1 -> Mux3/1
  enth/1 -> Mux3/2
  AH/1 -> Mux3/3
  Mux3/1 -> S-Function/1
  S-Function/1 -> Demux/1
  Demux/3 -> RH/1
  Demux/1 -> tempr/1
  Demux/2 -> Terminator/1

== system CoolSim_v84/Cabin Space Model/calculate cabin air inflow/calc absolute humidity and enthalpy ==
  note: mix u spec
  note: p/rho mix
  note: mix density
  press : Inport
  tempr : Inport  Port=2
  RH : Inport  Port=3
  Gain : Gain  Gain=cv_air
  Mux : Mux  Inputs=3
  Mux1 : Mux  Inputs=2
  Product : Product
  Sum : Sum  Inputs=++|
  Sum1 : Sum  Inputs=+|+
  add : Sum
  air int energy : Product
  calc abs humidity : Fcn  Expr=0.622*u(3)*u(2)/(u(1) - u(3)*u(2))
  calc h2o vapor u spec : Fcn  Expr=(2501.3+1.82*(u(1)-273.16))*1000.-r_h2o*u(1)
  calc psat_h2o : Fcn  Expr=exp(c08/u(1)+c09+c10*u(1)+c11*u(1)*u(1)+c12*u(1)*u(1)*u(1)+c13*log(u(1)))
  calc pure air density : Fcn  Expr=u(1)/rair/u(2)
  div : Product  Inputs=/*
  div1 : Product  Inputs=/*
  h2o density : Product
  h2o int energy : Product
  one : Constant  Value=1.0
  AH : Outport
  enth : Outport  Port=2
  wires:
  tempr/1 -> calc psat_h2o/1, Mux1/2, Gain/1, calc h2o vapor u spec/1
  RH/1 -> Mux/3
  press/1 -> Mux/1, Mux1/1, div1/2
  Mux/1 -> calc abs humidity/1
  calc psat_h2o/1 -> Mux/2
  Mux1/1 -> calc pure air density/1
  calc pure air density/1 -> air int energy/1, h2o density/2, Product/2
  calc abs humidity/1 -> AH/1, h2o density/1, Sum/1
  air int energy/1 -> Sum1/1
  Gain/1 -> air int energy/2
  h2o int energy/1 -> Sum1/2
  h2o density/1 -> h2o int energy/1
  calc h2o vapor u spec/1 -> h2o int energy/2
  div1/1 -> add/2
  add/1 -> enth/1
  div/1 -> add/1
  Sum/1 -> Product/1
  one/1 -> Sum/2
  Product/1 -> div/1, div1/1
  Sum1/1 -> div/2

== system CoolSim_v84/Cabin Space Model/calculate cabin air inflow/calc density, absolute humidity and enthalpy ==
  note: density
  note: specific enthalpy
  note: abs humidity
  note: mix u spec
  note: p/rho mix
  press : Inport
  tempr : Inport  Port=2
  RH : Inport  Port=3
  Gain : Gain  Gain=cv_air
  Gain1 : Gain  Gain=0.01
  Mux : Mux  Inputs=3
  Mux1 : Mux  Inputs=2
  Mux2 : Mux  Inputs=3
  Product : Product
  Sum : Sum  Inputs=++|
  Sum1 : Sum  Inputs=+|+
  Sum2 : Sum  Inputs=-+|
  add : Sum
  air int energy : Product
  calc abs humidity : Fcn  Expr=0.622*u(3)*u(2)/(u(1) - u(3)*u(2))
  calc h2o vapor u spec : Fcn  Expr=(2501.3+1.82*(u(1)-273.16))*1000.-r_h2o*u(1)
  calc psat_h2o : Fcn  Expr=exp(c08/u(1)+c09+c10*u(1)+c11*u(1)*u(1)+c12*u(1)*u(1)*u(1)+c13*log(u(1)))
  calc pure air density : Fcn  Expr=u(1)/rair/u(2)
  div : Product  Inputs=/*
  div1 : Product  Inputs=/*
  h2o density : Product
  h2o int energy : Product
  one : Constant  Value=1.0
  p h2o : Fcn  Expr=u(2)*u(3)
  dens : Outport
  AH : Outport  Port=2
  enth : Outport  Port=3
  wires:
  tempr/1 -> calc psat_h2o/1, Mux1/2, Gain/1, calc h2o vapor u spec/1
  RH/1 -> Gain1/1
  press/1 -> Mux/1, div1/2, Sum2/2
  Mux/1 -> calc abs humidity/1, p h2o/1
  calc psat_h2o/1 -> Mux/2
  Mux1/1 -> calc pure air density/1
  calc pure air density/1 -> air int energy/1, h2o density/2, Product/2
  calc abs humidity/1 -> Sum/1, h2o density/1, AH/1, Mux2/3
  Sum/1 -> Product/1
  one/1 -> Sum/2
  Product/1 -> dens/1, div/1, Mux2/1, div1/1
  air int energy/1 -> Sum1/1
  Gain/1 -> air int energy/2
  h2o int energy/1 -> Sum1/2
  h2o density/1 -> h2o int energy/1
  calc h2o vapor u spec/1 -> h2o int energy/2
  Mux2/1 -> [ambextras]
  Gain1/1 -> Mux/3
  Sum1/1 -> div/2
  div/1 -> add/1
  div1/1 -> add/2
  add/1 -> enth/1, Mux2/2
  Sum2/1 -> Mux1/1
  p h2o/1 -> Sum2/1

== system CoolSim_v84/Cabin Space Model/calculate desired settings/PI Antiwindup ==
  note: changed lower saturation limit to keep air always moving
  err : Inport
  I : Gain  Gain=f2_blowcontr
  Integrator : Integrator  InitialCondition=init_picontr1
  K : Gain  Gain=f1_blowcontr
  Ka : Gain  Gain=10
  Saturation : Saturate  UpperLimit=1  LowerLimit=0.2
  Sum1 : Sum  Inputs=|+-
  Sum2 : Sum  Inputs=++|
  Sum3 : Sum  Inputs=+-|
  contr1 : ToWorkspace  VariableName=contr1  SampleTime=-1
  contr2 : ToWorkspace  VariableName=contr2  SampleTime=-1
  contr3 : ToWorkspace  VariableName=contr3  SampleTime=-1
  contr4 : ToWorkspace  VariableName=contr4  SampleTime=-1
  cntrl : Outport
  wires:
  Saturation/1 -> Sum3/2, cntrl/1
  K/1 -> Sum2/1, contr2/1, Sum1/1
  Sum1/1 -> I/1
  I/1 -> Integrator/1
  Integrator/1 -> [picontr1], Sum2/2
  Sum2/1 -> Sum3/1, contr4/1, Saturation/1
  Sum3/1 -> Ka/1
  Ka/1 -> contr3/1, Sum1/2
  err/1 -> contr1/1, K/1

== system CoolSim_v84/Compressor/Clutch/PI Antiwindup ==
  note: introduce minimum RPM
  err : Inport
  trig : Inport  Port=2
  Clock : Clock
  Fcn1 : Fcn  Expr=u(2)+0.01-u(1)
  I : Gain  Gain=f2_comprcontr
  Integrator : Integrator  ExternalReset=rising  InitialConditionSource=external  InitialCondition=init_picontr2
  K : Gain  Gain=f1_comprcontr
  Ka : Gain  Gain=2
  Mux : Mux  Inputs=2
  Saturation : Saturate  UpperLimit=1.0  LowerLimit=rpm_minmaxrat
  Sum1 : Sum  Inputs=|+-
  Sum2 : Sum  Inputs=++|
  Sum3 : Sum  Inputs=+-|
  Sum4 : Sum  Inputs=|+-
  Switch : Switch  Threshold=deltat
  contr5 : ToWorkspace  VariableName=contr5  SampleTime=-1
  contr6 : ToWorkspace  VariableName=contr6  SampleTime=-1
  contr7 : ToWorkspace  VariableName=contr7  SampleTime=-1
  contr8 : ToWorkspace  VariableName=contr8  SampleTime=-1
  min to max rpm ratio : Constant  Value=rpm_minmaxrat
  one : Constant  Value=1.0
  one1 : Constant  Value=init_picontr2
  cntrl : Outport
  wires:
  one1/1 -> Switch/3
  Clock/1 -> Switch/2
  Switch/1 -> Integrator/3
  Fcn1/1 -> Switch/1
  one/1 -> Sum4/2
  Sum4/1 -> Integrator/2
  trig/1 -> Sum4/1
  min to max rpm ratio/1 -> Mux/2
  Mux/1 -> Fcn1/1
  Saturation/1 -> Sum3/2, cntrl/1
  K/1 -> Mux/1, Sum2/1, contr6/1, Sum1/1
  Sum1/1 -> I/1
  I/1 -> Integrator/1
  Integrator/1 -> [picontr2], Sum2/2
  Sum2/1 -> Sum3/1, contr8/1, Saturation/1
  Sum3/1 -> Ka/1
  Ka/1 -> contr7/1, Sum1/2
  err/1 -> contr5/1, K/1

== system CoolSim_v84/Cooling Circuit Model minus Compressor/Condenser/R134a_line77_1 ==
  note: qmd, hmd
  note: qmu, hmu
  pTrhu : Inport
  pTrhd : Inport  Port=2
  S-Function : S-Function  FunctionName=R134a_line77  Parameters=nparch, length, achan, pchan, relrough, mwall, cpwall, qcfactor, wplate, gappl, lfin, tp, thfin, densfin, lp, lw, theta, c1, c2, c3, c4, c5, nseg, damping, inmeth, m0, temp0, relerr, itmx, dgns, deltat  EnableBusSupport=off
  Terminator : Terminator
  Terminator1 : Terminator
  make md,hd,fi vector : Subsystem
  phvec_cond1 : Scope
  select hx rate : Fcn  Expr=u(1)
  qmhu : Outport
  qmhd : Outport  Port=2
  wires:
  S-Function/4 -> select hx rate/1
  S-Function/6 -> Terminator1/1
  S-Function/5 -> Terminator/1
  [condair1] -> make md,hd,fi vector/1(vT)
  S-Function/1 -> qmhu/1
  S-Function/2 -> phvec_cond1/1
  pTrhu/1 -> S-Function/1
  [initcond1] -> S-Function/2
  make md,hd,fi vector/1(mdhdfvec) -> S-Function/3
  pTrhd/1 -> S-Function/4
  S-Function/3 -> [mietcond1]
  S-Function/7 -> qmhd/1
  select hx rate/1 -> [qwrcond1]

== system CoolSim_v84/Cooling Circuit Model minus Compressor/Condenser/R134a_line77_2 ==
  note: qmd, hmd
  note: qmu, hmu
  pTrhu : Inport
  pTrhd : Inport  Port=2
  S-Function : S-Function  FunctionName=R134a_line77  Parameters=nparch, length, achan, pchan, relrough, mwall, cpwall, qcfactor, wplate, gappl, lfin, tp, thfin, densfin, lp, lw, theta, c1, c2, c3, c4, c5, nseg, damping, inmeth, m0, temp0, relerr, itmx, dgns, deltat  EnableBusSupport=off
  Terminator : Terminator
  Terminator1 : Terminator
  make md,hd,fi vector : Subsystem
  phvec_cond2 : Scope
  select hx rate : Fcn  Expr=u(1)
  qmhu : Outport
  qmhd : Outport  Port=2
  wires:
  select hx rate/1 -> [qwrcond2]
  S-Function/4 -> select hx rate/1
  S-Function/6 -> Terminator1/1
  S-Function/5 -> Terminator/1
  [condair1] -> make md,hd,fi vector/1(vT)
  S-Function/1 -> qmhu/1
  S-Function/2 -> phvec_cond2/1
  pTrhu/1 -> S-Function/1
  [initcond2] -> S-Function/2
  make md,hd,fi vector/1(mdhdfvec) -> S-Function/3
  pTrhd/1 -> S-Function/4
  S-Function/3 -> [mietcond2]
  S-Function/7 -> qmhd/1

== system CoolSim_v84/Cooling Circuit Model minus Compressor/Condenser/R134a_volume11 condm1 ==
  note: number of messages
  note: p, T, rho, h liquid phase
  qu : Inport
  "V, dVdt" : Inport  Port=2
  Hout : Inport  Port=3
  qd : Inport  Port=4
  S-Function : S-Function  FunctionName=R134a_volume11  Parameters=vol0, p0, tmp0, hspec0, lvf0, relerr, itmx, dgns  EnableBusSupport=off
  Terminator : Terminator
  Terminator1 : Terminator
  Terminator2 : Terminator
  ptrh_mix : Outport
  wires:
  qu/1 -> S-Function/1
  S-Function/1 -> ptrh_mix/1
  "V, dVdt"/1 -> S-Function/2
  Hout/1 -> S-Function/3
  qd/1 -> S-Function/4
  S-Function/5 -> Terminator/1
  S-Function/4 -> [lvfcondm1]
  S-Function/2 -> Terminator1/1
  S-Function/3 -> Terminator2/1

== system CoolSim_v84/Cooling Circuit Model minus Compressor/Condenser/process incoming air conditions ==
  note: air velocity due to fan
  note: Simplistic fan power calculation
  note: tempr in
  note: abs. humidity
  note: density
  note: area
  note: velocity
  note: mass flow rate
  note: pin
  note: pout
  note: relhumin
  Divide : Product  Inputs=****/
  Fcn1 : Fcn  Expr=u(3)
  Fcn3 : Fcn  Expr=u(1)+dpair_cond
  Fcn4 : Fcn  Expr=u(1)
  Gain : Gain  Gain=k_ram
  Mux1 : Mux  Inputs=5
  Product : Product  Inputs=3
  Sum : Sum  Inputs=++|
  Switch : Switch  Threshold=0.5
  Terminator1 : Terminator
  air in tempr : Constant  Value=tairin_cond
  air velocity : Constant  Value=vairin_cond
  "calc density, rel humidity and enthalpy" : Subsystem
  efficiency : Constant  Value=eff_fan
  flow area per plate : Constant  Value=aperp_cond
  flow area per plate1 : Constant  Value=aperp_cond
  minimum air velocity : Constant  Value=vairinmin_cond
  number of plates : Constant  Value=nc1+nc2
  pressure drop : Constant  Value=100.
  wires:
  flow area per plate1/1 -> Divide/4
  efficiency/1 -> Divide/5
  [fanonoff] -> Switch/2
  Sum/1 -> Product/1
  Gain/1 -> Sum/1
  Switch/1 -> Divide/1, Sum/2
  minimum air velocity/1 -> Switch/3
  air velocity/1 -> Switch/1
  [velvechicle] -> Gain/1
  "calc density, rel humidity and enthalpy"/3(enth) -> Terminator1/1
  Fcn3/1 -> Mux1/3, "calc density, rel humidity and enthalpy"/1(press)
  "calc density, rel humidity and enthalpy"/2(RH) -> Mux1/5
  "calc density, rel humidity and enthalpy"/1(dens) -> Product/2
  air in tempr/1 -> Mux1/2, "calc density, rel humidity and enthalpy"/2(tempr)
  [ambxtra] -> Fcn1/1
  Fcn1/1 -> "calc density, rel humidity and enthalpy"/3(AH)
  Divide/1 -> [pwfan]
  pressure drop/1 -> Divide/2
  number of plates/1 -> Divide/3
  [ambient] -> Fcn3/1, Fcn4/1
  flow area per plate/1 -> Product/3
  Product/1 -> Mux1/1
  Fcn4/1 -> Mux1/4
  Mux1/1 -> [condair1]

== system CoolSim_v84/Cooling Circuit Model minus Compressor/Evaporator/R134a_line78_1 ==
  note: qmu, hmu
  note: qmd, hmd
  note: p_out
  note: p_in
  pTrhu : Inport
  pTrhd : Inport  Port=2
  Mux1 : Mux  Inputs=2
  Mux3 : Mux  Inputs=2
  S-Function : S-Function  FunctionName=R134a_line78c  Parameters=nparch, length, achan, pchan, relrough, mwall, cpwall, qcfactor, wplate, gappl, lfin, tp, thfin, densfin, lp, lw, theta, c1, c2, c3, c4, c5, nseg, damping, inmeth, m0, temp0, relerr, itmx, dgns, deltat  EnableBusSupport=off
  S-Function2 : S-Function  FunctionName=airmixout01  Parameters=nseg, relerr, itmx, dgns  EnableBusSupport=off
  Terminator1 : Terminator
  Terminator4 : Terminator
  air out pressure : Constant  Value=p_ambient
  phvec_evap1 : Scope
  select hx rate : Fcn  Expr=u(1)
  qmhu : Outport
  qmhd : Outport  Port=2
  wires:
  select hx rate/1 -> [qwrevap1]
  air out pressure/1 -> Mux1/2, Mux3/2, S-Function2/2
  [airout_evap3] -> Mux1/1
  S-Function/7 -> qmhd/1
  S-Function/3 -> [mietevap1]
  pTrhd/1 -> S-Function/4
  Mux1/1 -> S-Function/3
  [initevap1] -> S-Function/2
  pTrhu/1 -> S-Function/1
  S-Function/2 -> phvec_evap1/1
  S-Function/1 -> qmhu/1
  S-Function/5 -> Mux3/1
  S-Function/6 -> Terminator1/1
  S-Function/4 -> select hx rate/1
  Mux3/1 -> S-Function2/1
  S-Function2/1 -> [airout_evap1]
  S-Function2/2 -> Terminator4/1

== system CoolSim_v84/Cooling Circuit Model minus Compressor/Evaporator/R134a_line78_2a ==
  note: qmu, hmu
  note: qmd, hmd
  note: p_out
  pTrhu : Inport
  pTrhd : Inport  Port=2
  Mux1 : Mux  Inputs=2
  Mux3 : Mux  Inputs=2
  S-Function : S-Function  FunctionName=R134a_line78c  Parameters=nparch, length, achan, pchan, relrough, mwall, cpwall, qcfactor, wplate, gappl, lfin, tp, thfin, densfin, lp, lw, theta, c1, c2, c3, c4, c5, nseg, damping, inmeth, m0, temp0, relerr, itmx, dgns, deltat  EnableBusSupport=off
  S-Function1 : S-Function  FunctionName=reverse_signal01  Parameters=nseg_evap3  EnableBusSupport=off
  S-Function2 : S-Function  FunctionName=airmixout01  Parameters=nseg, relerr, itmx, dgns  EnableBusSupport=off
  Terminator1 : Terminator
  Terminator4 : Terminator
  air out pressure : Constant  Value=p_ambient
  phvec_evap2a : Scope
  select hx rate : Fcn  Expr=u(1)
  qmhu : Outport
  qmhd : Outport  Port=2
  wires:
  air out pressure/1 -> Mux1/2, S-Function2/2, Mux3/2
  select hx rate/1 -> [qwrevap2a]
  [airout_evap3] -> S-Function1/1
  S-Function/7 -> qmhd/1
  S-Function/3 -> [mietevap2a]
  pTrhd/1 -> S-Function/4
  Mux1/1 -> S-Function/3
  [initevap2a] -> S-Function/2
  pTrhu/1 -> S-Function/1
  S-Function/2 -> phvec_evap2a/1
  S-Function/1 -> qmhu/1
  S-Function/5 -> Mux3/1
  S-Function/6 -> Terminator1/1
  S-Function/4 -> select hx rate/1
  S-Function1/1 -> Mux1/1
  Mux3/1 -> S-Function2/1
  S-Function2/1 -> [airout_evap2a]
  S-Function2/2 -> Terminator4/1

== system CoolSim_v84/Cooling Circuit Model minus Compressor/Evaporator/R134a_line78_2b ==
  note: qmu, hmu
  note: qmd, hmd
  note: p_out
  note: p_in
  pTrhu : Inport
  pTrhd : Inport  Port=2
  Mux1 : Mux  Inputs=2
  Mux3 : Mux  Inputs=2
  S-Function : S-Function  FunctionName=R134a_line78c  Parameters=nparch, length, achan, pchan, relrough, mwall, cpwall, qcfactor, wplate, gappl, lfin, tp, thfin, densfin, lp, lw, theta, c1, c2, c3, c4, c5, nseg, damping, inmeth, m0, temp0, relerr, itmx, dgns, deltat  EnableBusSupport=off
  S-Function2 : S-Function  FunctionName=airmixout01  Parameters=nseg, relerr, itmx, dgns  EnableBusSupport=off
  Terminator1 : Terminator
  Terminator4 : Terminator
  air out pressure : Constant  Value=p_ambient
  phvec_evap2b : Scope
  select hx rate : Fcn  Expr=u(1)
  qmhu : Outport
  qmhd : Outport  Port=2
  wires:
  air out pressure/1 -> Mux1/2, Mux3/2, S-Function2/2
  select hx rate/1 -> [qwrevap2b]
  [airout_evap4] -> Mux1/1
  S-Function/7 -> qmhd/1
  S-Function/3 -> [mietevap2b]
  pTrhd/1 -> S-Function/4
  Mux1/1 -> S-Function/3
  [initevap2b] -> S-Function/2
  pTrhu/1 -> S-Function/1
  S-Function/2 -> phvec_evap2b/1
  S-Function/1 -> qmhu/1
  S-Function/5 -> Mux3/1
  S-Function/6 -> Terminator1/1
  S-Function/4 -> select hx rate/1
  Mux3/1 -> S-Function2/1
  S-Function2/1 -> [airout_evap2b]
  S-Function2/2 -> Terminator4/1

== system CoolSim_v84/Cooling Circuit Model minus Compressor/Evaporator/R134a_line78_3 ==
  note: qmu, hmu
  note: qmd, hmd
  pTrhu : Inport
  pTrhd : Inport  Port=2
  Fcn1 : Fcn  Expr=(u(32)+u(33)+u(34)+u(35)+u(36)+u(37)+u(38)+u(39)+u(40)+u(41))/10.0
  Fcn4 : Fcn  Expr=u(4)
  Mux2 : Mux  Inputs=2
  S-Function : S-Function  FunctionName=R134a_line78c  Parameters=nparch, length, achan, pchan, relrough, mwall, cpwall, qcfactor, wplate, gappl, lfin, tp, thfin, densfin, lp, lw, theta, c1, c2, c3, c4, c5, nseg, damping, inmeth, m0, temp0, relerr, itmx, dgns, deltat  EnableBusSupport=off
  Terminator1 : Terminator
  make vectors : Subsystem
  phvec_evap3 : Scope
  select hx rate : Fcn  Expr=u(1)
  qmhu : Outport
  qmhd : Outport  Port=2
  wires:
  Fcn4/1 -> Mux2/2
  [evapair] -> Fcn4/1, make vectors/1(mdtppf)
  make vectors/1(vector) -> S-Function/3
  select hx rate/1 -> [qwrevap3]
  Mux2/1 -> [airout_evap3]
  S-Function/7 -> qmhd/1
  S-Function/3 -> Fcn1/1, [mietevap3]
  pTrhd/1 -> S-Function/4
  [initevap3] -> S-Function/2
  pTrhu/1 -> S-Function/1
  S-Function/2 -> phvec_evap3/1
  S-Function/1 -> qmhu/1
  S-Function/5 -> Mux2/1
  S-Function/6 -> Terminator1/1
  S-Function/4 -> select hx rate/1
  Fcn1/1 -> [twallevap]

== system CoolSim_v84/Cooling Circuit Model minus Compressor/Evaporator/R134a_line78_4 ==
  note: qmu, hmu
  note: qmd, hmd
  pTrhu : Inport
  pTrhd : Inport  Port=2
  Fcn4 : Fcn  Expr=u(4)
  Mux2 : Mux  Inputs=2
  S-Function : S-Function  FunctionName=R134a_line78c  Parameters=nparch, length, achan, pchan, relrough, mwall, cpwall, qcfactor, wplate, gappl, lfin, tp, thfin, densfin, lp, lw, theta, c1, c2, c3, c4, c5, nseg, damping, inmeth, m0, temp0, relerr, itmx, dgns, deltat  EnableBusSupport=off
  Terminator1 : Terminator
  make vectors : Subsystem
  phvec_evap4 : Scope
  select hx rate : Fcn  Expr=u(1)
  select1 : Fcn  Expr=u(1)
  qmhu : Outport
  qmhd : Outport  Port=2
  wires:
  select1/1 -> [td_evap]
  Fcn4/1 -> Mux2/2
  [evapair] -> Fcn4/1, make vectors/1(mdtppf)
  make vectors/1(vector) -> S-Function/3
  select hx rate/1 -> [qwrevap4]
  Mux2/1 -> [airout_evap4]
  S-Function/7 -> qmhd/1
  S-Function/3 -> [mietevap4]
  pTrhd/1 -> S-Function/4
  [initevap4] -> S-Function/2
  pTrhu/1 -> S-Function/1
  S-Function/2 -> phvec_evap4/1
  S-Function/1 -> qmhu/1
  S-Function/5 -> Mux2/1
  S-Function/6 -> select1/1, Terminator1/1
  S-Function/4 -> select hx rate/1

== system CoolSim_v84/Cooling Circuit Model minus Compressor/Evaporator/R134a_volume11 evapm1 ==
  note: p, T, rho, h vapor phase
  note: p, T, rho, h liquid phase
  note: number of messages
  qu : Inport
  "V, dVdt" : Inport  Port=2
  Hout : Inport  Port=3
  qd : Inport  Port=4
  S-Function : S-Function  FunctionName=R134a_volume11  Parameters=vol0, p0, tmp0, hspec0, lvf0, relerr, itmx, dgns  EnableBusSupport=off
  Terminator : Terminator
  Terminator1 : Terminator
  Terminator2 : Terminator
  ptrh_mix : Outport
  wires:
  S-Function/4 -> [lvfevapm1]
  S-Function/3 -> Terminator1/1
  S-Function/2 -> Terminator/1
  S-Function/5 -> Terminator2/1
  qd/1 -> S-Function/4
  Hout/1 -> S-Function/3
  "V, dVdt"/1 -> S-Function/2
  S-Function/1 -> ptrh_mix/1
  qu/1 -> S-Function/1

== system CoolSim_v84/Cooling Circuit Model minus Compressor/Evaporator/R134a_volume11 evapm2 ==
  note: p, T, rho, h vapor phase
  note: p, T, rho, h liquid phase
  note: number of messages
  qu : Inport
  "V, dVdt" : Inport  Port=2
  Hout : Inport  Port=3
  qd : Inport  Port=4
  S-Function : S-Function  FunctionName=R134a_volume11  Parameters=vol0, p0, tmp0, hspec0, lvf0, relerr, itmx, dgns  EnableBusSupport=off
  Terminator : Terminator
  Terminator1 : Terminator
  Terminator2 : Terminator
  ptrh_mix : Outport
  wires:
  S-Function/4 -> [lvfevapm2]
  S-Function/3 -> Terminator1/1
  S-Function/2 -> Terminator/1
  S-Function/5 -> Terminator2/1
  qd/1 -> S-Function/4
  Hout/1 -> S-Function/3
  "V, dVdt"/1 -> S-Function/2
  S-Function/1 -> ptrh_mix/1
  qu/1 -> S-Function/1

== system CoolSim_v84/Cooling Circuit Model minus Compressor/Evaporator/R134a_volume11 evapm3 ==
  note: p, T, rho, h vapor phase
  note: p, T, rho, h liquid phase
  note: number of messages
  qu : Inport
  "V, dVdt" : Inport  Port=2
  Hout : Inport  Port=3
  qd : Inport  Port=4
  S-Function : S-Function  FunctionName=R134a_volume11  Parameters=vol0, p0, tmp0, hspec0, lvf0, relerr, itmx, dgns  EnableBusSupport=off
  Terminator : Terminator
  Terminator1 : Terminator
  Terminator2 : Terminator
  ptrh_mix : Outport
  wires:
  S-Function/4 -> [lvfevapm3]
  S-Function/3 -> Terminator1/1
  S-Function/2 -> Terminator/1
  S-Function/5 -> Terminator2/1
  qd/1 -> S-Function/4
  Hout/1 -> S-Function/3
  "V, dVdt"/1 -> S-Function/2
  S-Function/1 -> ptrh_mix/1
  qu/1 -> S-Function/1
